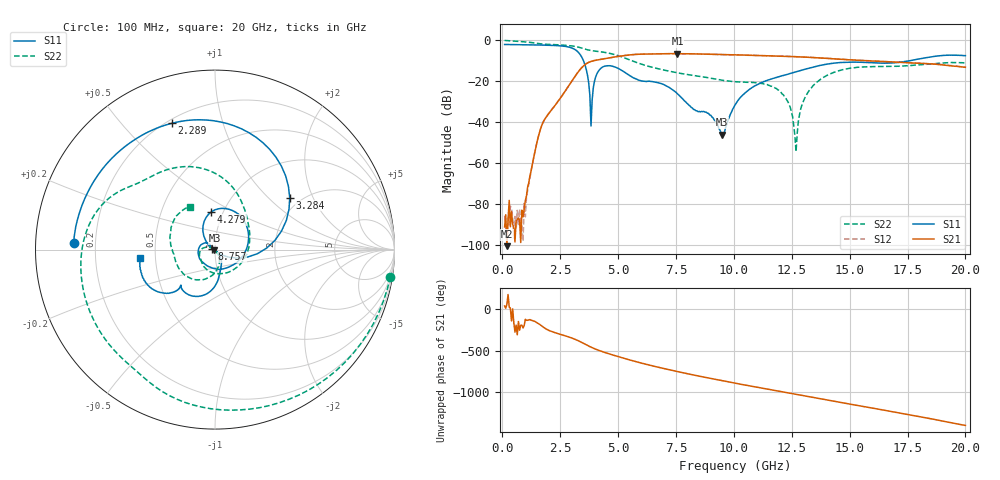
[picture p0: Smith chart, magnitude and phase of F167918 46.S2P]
!  2-Port S-parameters saved by WinCal
! VAR MeasName=S-Parameters (CALIBRATED_DATA) read from VNA (N5242A)
! VAR MeasDate=2016-11-22 10:27:01
! VAR NAME=F167918 46
! VAR FILENAME=F167918 46.S2P
! VAR DATE=2016-11-22 10:27:01
! VAR PHYS_PORTS=1,2
# Hz S DB R 50
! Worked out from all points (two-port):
!   401 points, 100 MHz to 20 GHz, reference 50 ohm
!   highest |S21| = -6.54 dB at 7.562 GHz (marker M1); lowest = -100.8 dB at 199.5 MHz (marker M2)
!   |S21| within 3 dB of the highest: 4.157 GHz to 14.92 GHz (10.77 GHz wide, 113 % of centre)
!   lowest |S11| = -46.2 dB at 9.503 GHz (marker M3), VSWR 1.01, Z = 49.7 - j0.401 ohm
!   |S11| at or under -10 dB: 3.504 GHz to 17.61 GHz (14.1 GHz wide, 134 % of centre)
!   |S22| runs from -54.6 to -0.1 dB; largest |S21 - S12| = 0.0065
!   S11 on the Smith chart (normalised r, x): 100 MHz: 0.12, +0.02; 2.289 GHz: 0.22, +0.69; 3.284 GHz: 1.75, +1.37; 4.279 GHz: 0.88, +0.39; 8.757 GHz: 0.97, +0.00; 20 GHz: 0.41, -0.05
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1e8  -2.06 177.3  -91.36 40.4  -85.84 -104.5  -0.10 -8.8
1.995e8  -2.07 174.6  -100.78 60.2  -97.08 -109.2  -0.16 -17.0
9.4575e8  -2.19 154.6  -82.44 164.8  -79.81 -151.1  -0.77 -74.3
1.64225e9  -2.34 133.7  -43.67 171.2  -43.69 170.2  -1.75 -118.6
2.289e9  -2.57 109.0  -31.70 76.5  -31.65 76.3  -2.15 -150.9
3.284e9  -5.89 34.8  -15.41 -19.9  -15.42 -19.8  -3.36 158.8
3.43325e9  -8.29 15.6  -13.37 -40.5  -13.37 -40.4  -3.83 151.8
3.83125e9  -42.01 -100.5  -10.38 -96.9  -10.35 -97.0  -5.03 137.7
4.279e9  -13.52 95.7  -9.31 -147.0  -9.29 -147.3  -5.68 121.3
5.62225e9  -18.13 -52.0  -7.05 99.5  -7.04 99.4  -10.14 62.6
6.7665e9  -20.88 174.9  -6.59 18.7  -6.60 18.5  -14.03 14.1
7.5625e9  -26.16 136.1  -6.54 -31.3  -6.58 -31.4  -15.92 -34.0
8.7565e9  -35.17 174.5  -6.77 -101.0  -6.77 -101.0  -18.12 -105.4
9.50275e9  -46.15 -125.0  -6.96 -141.9  -6.98 -142.0  -19.55 -132.8
1.005e10  -31.65 -47.6  -7.12 -171.2  -7.14 -171.1  -20.32 -144.3
1.19405e10  -17.89 -77.7  -7.80 90.9  -7.76 90.9  -24.51 169.0
1.238825e10  -16.42 -81.3  -7.95 68.0  -7.91 68.0  -31.57 155.0
1.268675e10  -15.42 -84.0  -8.05 52.7  -8.04 52.7  -54.56 -107.2
1.338325e10  -13.26 -92.6  -8.43 17.0  -8.38 17.2  -22.78 -70.1
1.51245e10  -10.69 -122.7  -9.64 -69.5  -9.57 -69.7  -13.53 -130.7
1.67165e10  -11.17 -133.6  -10.51 -148.1  -10.50 -148.3  -12.81 -167.4
2e10  -7.52 -173.3  -13.24 38.7  -13.20 38.0  -11.14 120.2
